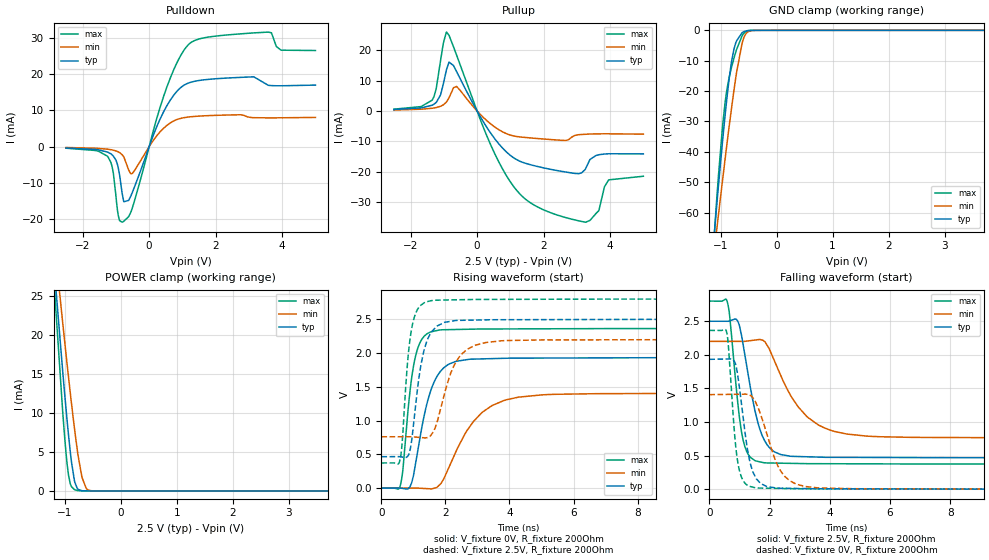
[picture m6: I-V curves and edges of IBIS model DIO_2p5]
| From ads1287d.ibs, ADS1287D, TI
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|   Model
[Model]   DIO_2p5
Model_type   I/O
Polarity   Non-Inverting
Enable   Active-Low
Vinl = 0.75
Vinh = 1.75
Vmeas = 1.25
Vref = 0
Cref = 1pF
Rref = 100000
|   typ   min   max
C_comp   3.504pF   3.036pF   3.899p
[Voltage Range]   2.5   2.2   2.8
[Temperature Range]   27   125   -40
[Pullup Reference]   2.5   2.2   2.8
[Pulldown Reference]   0   0   -0
[Power Clamp Reference]   2.5   2.2   2.8
[GND Clamp Reference]   0   0   0
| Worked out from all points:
|   slope of the pulldown table from 0 to 0.375 V, typ, clamps not added: 44.2 ohm
|   slope of the pullup table from 0 to 0.375 V, typ, clamps not added: 55.4 ohm
|   GND clamp passes 1 mA (typ) near -0.62 V on its own axis
|   POWER clamp passes 1 mA (typ) near -0.81 V on its own axis
|   falling waveform, V_fixture 2.5V, R_fixture 200Ohm: 20-80 % time 550ps typ, 1.17ns min, 335ps max; typ from 2.5 V to 0.466 V
|   rising waveform, V_fixture 0V, R_fixture 200Ohm: 20-80 % time 549ps typ, 1.07ns min, 329ps max; typ from 0 V to 1.93 V
|   rising waveform, V_fixture 2.5V, R_fixture 200Ohm: 20-80 % time 377ps typ, 610ps min, 252ps max; typ from 0.466 V to 2.5 V
|   falling waveform, V_fixture 0V, R_fixture 200Ohm: 20-80 % time 370ps typ, 664ps min, 249ps max; typ from 1.93 V to 0 V
[Pulldown]
|   Voltage   I(typ)   I(min)   I(max)
-2.5V     -353uA     -224.1uA   -417.6uA
-1.24V    -1.524mA   -700.5uA   -2.764mA
-1.083V   -2.516mA   -951.2uA   -6.962mA
-977.5mV  -4.216mA   -1.238mA   -15.53mA
-812.5mV  -12.82mA   -2.205mA   -20.8mA
-760mV    -15.16mA   -2.848mA   -20.52mA
-512.5mV  -12.74mA   -7.38mA    -17.05mA
522.5mV   11.12mA    5.789mA    16.17mA
1.228V    17.68mA    8.219mA    28.49mA
3.583V    16.9mA     7.94mA     31.56mA
3.965V    16.77mA    7.958mA    26.58mA
5V        16.96mA    8.062mA    26.49mA
[GND Clamp]
|   Voltage   I(typ)   I(min)   I(max)
-2.5V     -399.4mA   -328.2mA   -471.2mA
-1.232V   -93.59mA   -92.92mA   -99.69mA
-1.067V   -57.42mA   -65.52mA   -55.36mA
-1.06V    -55.84mA   -64.32mA   -53.46mA
-962.5mV  -36.11mA   -49.05mA   -31.16mA
-917.5mV  -27.74mA   -42.2mA    -23.5mA
-805mV    -10.42mA   -25.77mA   -12.24mA
-715mV    -3.499mA   -13.99mA   -6.349mA
-580mV    -417uA     -2.255mA   -930.9uA
-505mV    -73.97uA   -428.2uA   -139.2uA
-347.5mV  -1.109uA   -10.57uA   -987.1nA
5V        0A         0A         0A
[Pullup]
|   Voltage   I(typ)   I(min)   I(max)
-2.5V     456.3uA    297.4uA    577.2uA
-1.353V   1.879mA    880.5uA    3.528mA
-1.105V   5.11mA     1.504mA    16.06mA
-917.5mV  13.67mA    2.981mA    25.97mA
-842.5mV  16.1mA     4.351mA    24.89mA
-617.5mV  12.99mA    8.068mA    18.45mA
537.5mV   -9.248mA   -5.346mA   -14.22mA
1.482V    -17.34mA   -8.776mA   -29.31mA
3.268V    -18.94mA   -7.691mA   -36.66mA
3.658V    -14.44mA   -7.548mA   -32.88mA
3.958V    -14.12mA   -7.539mA   -22.71mA
5V        -14.14mA   -7.65mA    -21.52mA
[POWER Clamp]
|   Voltage   I(typ)   I(min)   I(max)
-2.5V     152.2mA    129.3mA    183.1mA
-1.188V   28.48mA    32.1mA     26.31mA
-1.038V   15.43mA    21.62mA    10.28mA
-992.5mV  11.74mA    18.56mA    6.139mA
-955mV    8.823mA    16.06mA    3.296mA
-902.5mV  5.116mA    12.66mA    959.2uA
-820mV    1.112mA    7.651mA    151.2uA
-775mV    305uA      5.211mA    56.92uA
-692.5mV  25.36uA    1.758mA    9.93uA
-617.5mV  5.437uA    345.2uA    4.718uA
-542.5mV  3.212uA    46.65uA    4.119uA
5V        0A         0A         0A
[Ramp]
R_load = 200
|   typ   min   max
dV/dt_r   1.15982/5.45659e-10   0.844385/1.07026e-09   1.41818/3.27493e-10
dV/dt_f   1.22033/5.46467e-10   0.863282/1.15994e-09   1.45598/3.34603e-10
[Falling Waveform]
V_fixture = 2.5V
V_fixture_min = 2.2V
V_fixture_max = 2.8V
R_fixture = 200Ohm
C_fixture = 0F
|   Time   V(typ)   V(min)   V(max)
0s        2.5V       2.2V       2.8V
607ps     2.5V       2.2V       2.769V
960.2ps   2.485V     2.2V       1.219V
1.241ns   1.834V     2.204V     560.7mV
1.518ns   1.161V     2.22V      423.6mV
1.809ns   745.5mV    2.208V     393.9mV
2.369ns   515.5mV    1.694V     386.8mV
3.225ns   482.5mV    1.087V     380.1mV
5.213ns   472.4mV    790.5mV    377.1mV
50ns      466mV      761.1mV    373.3mV
[Rising Waveform]
V_fixture = 0V
V_fixture_min = 0V
V_fixture_max = 0V
R_fixture = 200Ohm
C_fixture = 0F
|   Time   V(typ)   V(min)   V(max)
0s        -433.5nV   561.5nV    -6.06nV
584.4ps   162.6uV    188.1uV    31.3mV
669.8ps   -4.525mV   215.5uV    273.5mV
899.8ps   29.04mV    289.4uV    1.465V
1.201ns   736.3mV    -1.373mV   2.153V
1.518ns   1.413V     -9.853mV   2.309V
1.809ns   1.707V     45.51mV    2.342V
3.124ns   1.914V     1.112V     2.357V
5.028ns   1.926V     1.382V     2.36V
50ns      1.933V     1.407V     2.364V
[Rising Waveform]
V_fixture = 2.5V
V_fixture_min = 2.2V
V_fixture_max = 2.8V
R_fixture = 200Ohm
C_fixture = 0F
|   Time   V(typ)   V(min)   V(max)
0s        466mV      761.1mV    373.3mV
562.3ps   465.6mV    761.1mV    386.6mV
646.1ps   460.7mV    761.1mV    666.4mV
857.6ps   504.2mV    761.1mV    2.066V
1.003ns   947.8mV    758.7mV    2.492V
1.229ns   1.811V     749.4mV    2.708V
1.614ns   2.339V     828.6mV    2.782V
2.422ns   2.485V     1.937V     2.79V
3.744ns   2.494V     2.182V     2.795V
50ns      2.5V       2.2V       2.8V
[Falling Waveform]
|Gnd
V_fixture = 0V
V_fixture_min = 0V
V_fixture_max = 0V
R_fixture = 200Ohm
C_fixture = 0F
|   Time   V(typ)   V(min)   V(max)
0s        1.933V     1.407V     2.364V
584.4ps   1.938V     1.411V     2.317V
857.6ps   1.877V     1.412V     717.1mV
957.2ps   1.649V     1.413V     365.8mV
1.068ns   1.266V     1.414V     177.4mV
1.327ns   445.8mV    1.403V     42.6mV
1.541ns   172.2mV    1.291V     18.9mV
2.422ns   13.84mV    235.5mV    10.28mV
3.641ns   6.142mV    18.4mV     5.471mV
50ns      -571nV     578.5nV    -45.97nV
